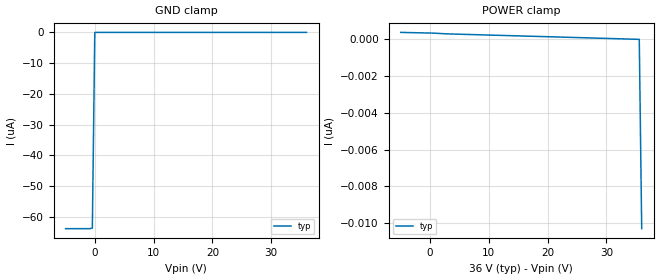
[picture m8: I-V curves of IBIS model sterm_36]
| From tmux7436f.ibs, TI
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| sterm_36
[Model]   sterm_36
Model_type   Terminator
|   typ   min   max
C_comp   4.014581e-12   NA   NA
[Voltage Range]   36   NA   NA
[Temperature Range]   27   NA   NA
[Power Clamp Reference]   36   NA   NA
[GND Clamp Reference]   0   NA   NA
[GND Clamp]
|   Voltage   I(typ)   I(min)   I(max)
-5V       -63.89uA   NA         NA
-444.4mV  -63.69uA   NA         NA
-30.3mV   -33.06nA   NA         NA
36V       320.1pA    NA         NA
[POWER Clamp]
|   Voltage   I(typ)   I(min)   I(max)
-5V       355.4pA    NA         NA
383.8mV   317.3pA    NA         NA
35.59V    -22.67pA   NA         NA
36V       -10.29nA   NA         NA
